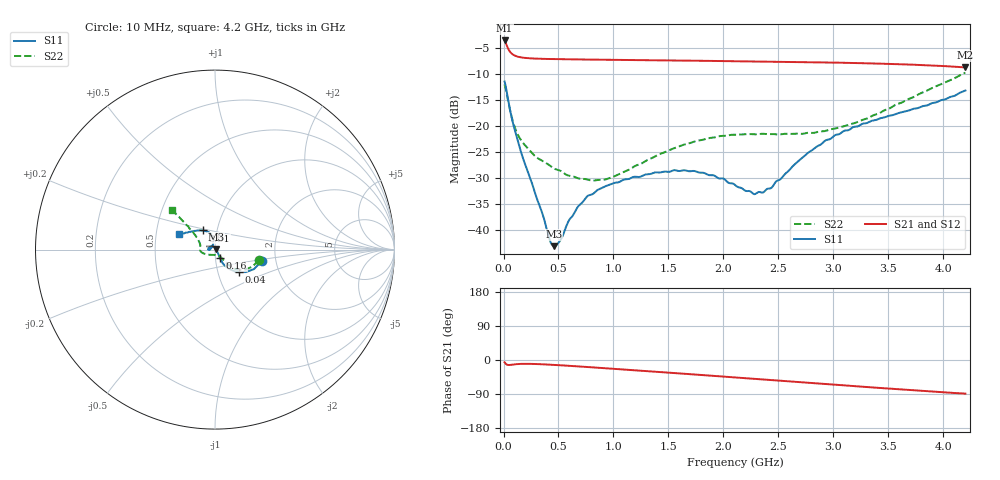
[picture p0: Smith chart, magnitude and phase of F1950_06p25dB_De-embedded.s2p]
! Integrated Device Technology
! Corporate Headquarters
! 6024 Silver Creek Valley Road
! San Jose, CA 95138  USA
! Phone:  1-408-284-8200
! Toll Free:  1-800-223-1366
! Webpage:  http://www.idt.com/
! Timing and RF Division
! 515 Groton Road, Suite 102
! Westford, MA 01886-6024
! Device:  F1950
! Description: 7-bit 0.25 dB Digital Step Attenuator
! Frequency:  150.0 -  4000.00 MHz
! Package:  4x4 mm Thin QFN Plastic Package: 24 pin
! Ports:  2 RF, 12 DC
!  Pin  1  = D0
!  Pin  2  = VDD
!  Pin  3  = Vmode
!  Pin  4  = GND
!  Pin  5  = RF1  =  Port 1
!  Pin  6  = GND
!  Pin  7  = GND
!  Pin  8  = GND
!  Pin  9  = GND
!  Pin 10  = GND
!  Pin 11  = GND
!  Pin 12  = GND
!  Pin 13  = GND
!  Pin 14  = RF2  =  Port 2
!  Pin 15  = GND
!  Pin 16  = LE
!  Pin 17  = CLK
!  Pin 18  = DATE
!  Pin 19  = D6
!  Pin 20  = D5
!  Pin 21  = D4
!  Pin 22  = D3
!  Pin 23  = D2
!  Pin 24  = D1
! State:  25
! Atten State:  6.25 dB
! Voltage:  +5.00 Volts
! Current:  Not Measured mA
! Data:  The device was measured on a the F195X evaluation board which has
!  individual transmission lines to the RF pins.  Data was collected
!  using a calibrated network analyzer.  The evaluation board was
!  de-embedded using a TRL calibration technique.
!  The reference plane is the edge of the package pin.
! Misc:  Board 2019
!  Action Tracker AT0250
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# GHz S dB R 50
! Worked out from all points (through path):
!   420 points, 10 MHz to 4.2 GHz, reference 50 ohm
!   highest |S21| = -3.51 dB at 10 MHz (marker M1); lowest = -8.7 dB at 4.2 GHz (marker M2)
!   group delay of S21, straight-line fit = 56.1 ps
!   lowest |S11| = -43.2 dB at 460 MHz (marker M3), VSWR 1.01, Z = 50.6 + j0.315 ohm
!   |S11| at or under -10 dB: start of sweep to end of sweep
!   |S22| runs from -30.5 to -9.7 dB; largest |S21 - S12| = 0.00058
!   S11 on the Smith chart (normalised r, x): 10 MHz: 1.69, -0.23; 40 MHz: 1.26, -0.33; 160 MHz: 1.05, -0.10; 3.51 GHz: 0.86, +0.19; 4.2 GHz: 0.65, +0.12
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0.01  -11.43 -13.7  -3.51 -6.1  -3.51 -6.1  -11.97 -13.8
0.04  -14.69 -42.9  -4.99 -13.0  -4.99 -13.1  -14.99 -39.5
0.1  -20.57 -59.8  -6.40 -11.5  -6.40 -11.5  -20.10 -49.1
0.16  -25.06 -60.4  -6.77 -10.3  -6.77 -10.3  -22.74 -51.3
0.29  -33.12 -48.7  -7.00 -10.6  -7.00 -10.6  -25.86 -53.2
0.42  -41.91 -5.4  -7.08 -12.3  -7.08 -12.3  -27.59 -56.2
0.46  -43.15 26.6  -7.10 -12.9  -7.10 -12.9  -28.18 -59.0
0.51  -42.24 65.3  -7.12 -13.8  -7.12 -13.8  -28.57 -61.8
0.59  -38.37 94.7  -7.14 -15.2  -7.14 -15.2  -29.54 -67.2
0.71  -34.86 113.5  -7.17 -17.5  -7.17 -17.5  -30.18 -78.4
0.77  -33.41 119.1  -7.19 -18.6  -7.19 -18.6  -30.36 -84.6
0.94  -31.49 133.9  -7.23 -22.0  -7.23 -22.0  -30.21 -106.6
1.41  -28.95 167.4  -7.34 -31.5  -7.34 -31.5  -25.49 -150.2
1.74  -28.68 -178.1  -7.41 -38.3  -7.41 -38.3  -22.95 -164.5
2.11  -31.44 176.2  -7.51 -46.1  -7.51 -46.1  -21.68 -175.8
2.28  -33.14 151.9  -7.55 -49.6  -7.55 -49.6  -21.60 179.7
2.36  -32.81 137.4  -7.57 -51.3  -7.57 -51.3  -21.50 177.5
2.44  -31.83 121.8  -7.59 -52.9  -7.59 -52.9  -21.53 175.3
2.81  -24.60 99.2  -7.70 -60.8  -7.70 -60.8  -21.33 162.3
3.1  -20.90 105.2  -7.81 -67.0  -7.81 -67.0  -20.02 153.1
3.51  -18.00 122.2  -8.03 -75.6  -8.02 -75.7  -16.61 142.7
4.2  -13.15 156.9  -8.71 -88.6  -8.71 -88.7  -9.72 137.5
